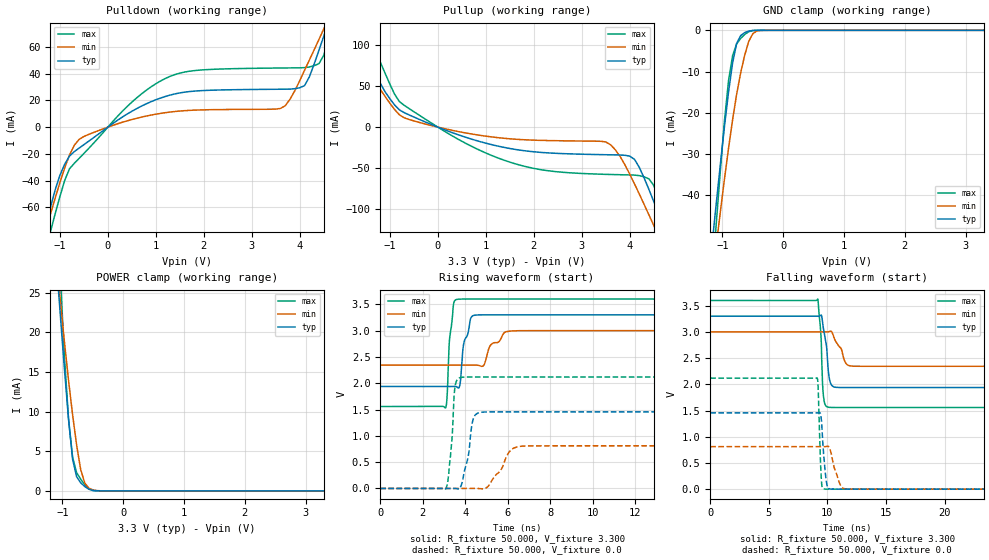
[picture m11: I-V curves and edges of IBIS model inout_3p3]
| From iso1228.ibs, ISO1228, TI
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|   Model inout_3p3
[Model] inout_3p3
Model_type I/O
Vinl =  0.990V
Vinh =  2.310V
Polarity   Non-Inverting
Enable   Active-High
Vmeas = 1.65
Vref = 0
Cref = 15pF
Rref = 1000
C_comp   0.978pF   1.050pF   0.889pF
[Model Spec]
Vinh   2.310V   2.100V   2.520V
Vinl   0.990V   0.900V   1.080V
[Temperature Range]   27.000   0.150k   -40.000
[Voltage Range]   3.300V   3.000V   3.600V
[Pullup Reference]   3.300V   3.000V   3.600V
[Pulldown Reference]   0.0V   0.0V   0.0V
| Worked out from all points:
|   slope of the pulldown table from 0 to 0.495 V, typ, clamps not added: 42.2 ohm
|   slope of the pullup table from 0 to 0.495 V, typ, clamps not added: 46.1 ohm
|   GND clamp passes 1 mA (typ) near -0.68 V on its own axis
|   POWER clamp passes 1 mA (typ) near -0.70 V on its own axis
|   rising waveform, R_fixture 50.000, V_fixture 3.300: 20-80 % time 356ps typ, 720ps min, 207ps max; typ from 1.94 V to 3.3 V
|   rising waveform, R_fixture 50.000, V_fixture 0.0: 20-80 % time 354ps typ, 726ps min, 215ps max; typ from 0 V to 1.46 V
|   falling waveform, R_fixture 50.000, V_fixture 3.300: 20-80 % time 412ps typ, 821ps min, 243ps max; typ from 3.3 V to 1.94 V
|   falling waveform, R_fixture 50.000, V_fixture 0.0: 20-80 % time 293ps typ, 603ps min, 185ps max; typ from 1.46 V to 0 V
[Pulldown]
|Voltage   I(typ)   I(min)   I(max)
-3.3V     -447.8mA   -372.8mA   -654.4mA
-1.3V     -74.39mA   -77.85mA   -94.82mA
-1.2V     -60.33mA   -65.41mA   -78.6mA
-900mV    -27.72mA   -30.46mA   -39.85mA
-600mV    -15.68mA   -9.201mA   -23.38mA
500mV     11.84mA    5.676mA    18.66mA
1.3V      23.95mA    11.27mA    37.96mA
3.6V      28.3mA     13.97mA    44.16mA
4.1V      31.01mA    42.51mA    44.42mA
4.5V      67.87mA    73.32mA    53.59mA
4.7V      89mA       89.09mA    81.73mA
6.6V      358.2mA    289.3mA    493.9mA
[Pullup]
|Voltage   I(typ)   I(min)   I(max)
-3.3V     356.7mA    258.7mA    567mA
-2.1V     161.1mA    122.4mA    246.9mA
-1.8V     121.5mA    96.5mA     180.5mA
-1.5V     87.45mA    71.23mA    126mA
-700mV    17.66mA    11.4mA     26.61mA
1.4V      -24.96mA   -13.72mA   -40.75mA
3.5V      -33.67mA   -18.07mA   -57.65mA
4.1V      -39.42mA   -69.47mA   -58.55mA
4.4V      -76.17mA   -107.2mA   -63.21mA
4.6V      -105.6mA   -132.9mA   -86.69mA
4.8V      -135.9mA   -159mA     -125.7mA
6.6V      -482.2mA   -443.3mA   -617.5mA
[GND_clamp]
|Voltage   I(typ)   I(min)   I(max)
-3.3V     -446.5mA   -372.3mA   -652.2mA
-1.167V   -51.36mA   -60.11mA   -59.79mA
-1.1V     -41.74mA   -51.92mA   -46.53mA
-1.033V   -32.37mA   -43.89mA   -33.74mA
-967mV    -23.36mA   -36.1mA    -21.98mA
-900mV    -15.01mA   -28.65mA   -12.25mA
-833mV    -7.919mA   -21.71mA   -6.137mA
-767mV    -3.23mA    -15.56mA   -3.327mA
-633mV    -537.4uA   -5.994mA   -992.5uA
-500mV    -36.13uA   -809.1uA   -56.28uA
-367mV    -1.312uA   -33.13uA   -1.236uA
3.3V      0A         0A         0A
[POWER_clamp]
|Voltage   I(typ)   I(min)   I(max)
-3.3V     327.5mA    237.7mA    524.4mA
-1.1V     28.87mA    29.08mA    37.17mA
-1.033V   22.02mA    23.87mA    26.91mA
-967mV    15.37mA    18.79mA    16.96mA
-900mV    9.079mA    13.99mA    9.126mA
-833mV    4.017mA    9.616mA    4.268mA
-767mV    1.792mA    5.817mA    2.311mA
-700mV    1.03mA     2.71mA     1.49mA
-633mV    556.9uA    1.007mA    803.4uA
-567mV    225.9uA    363.5uA    292.8uA
-300mV    7.304uA    7.368uA    10.1uA
3.3V      0A         0A         775.8nA
[Ramp]
| variable   typ   min   max
dV/dt_r   0.873/0.354n   0.487/0.726n   1.271/0.213n
dV/dt_f   0.817/0.414n   0.394/0.818n   1.225/0.244n
R_load = 50.000
[Rising Waveform]
R_fixture= 50.000
V_fixture= 3.300
V_fixture_min= 3.000
V_fixture_max= 3.600
|time   V(typ)   V(min)   V(max)
0s        1.938V     2.344V     1.558V
3.08ns    1.938V     2.344V     1.536V
3.15ns    1.938V     2.344V     1.809V
3.25ns    1.938V     2.344V     2.804V
3.43ns    1.939V     2.344V     3.455V
3.7ns     1.913V     2.344V     3.598V
3.94ns    2.78V      2.344V     3.6V
4.6ns     3.298V     2.342V     3.6V
6.49ns    3.3V       2.998V     3.6V
100ns     3.3V       3V         3.6V
[Rising Waveform]
R_fixture= 50.000
V_fixture= 0.0
V_fixture_min= 0.0
V_fixture_max= 0.0
|time   V(typ)   V(min)   V(max)
0s        258.3nV    99.06nV    1.22nV
3.08ns    1.462uV    99.06nV    -5.843mV
3.3ns     -36.21uV   95.06nV    611.5mV
3.53ns    798uV      169nV      1.972V
3.9ns     207.8mV    -2.457uV   2.116V
4.37ns    1.322V     198uV      2.118V
4.94ns    1.453V     187.2uV    2.118V
6.15ns    1.455V     733.5mV    2.118V
7.03ns    1.455V     809.6mV    2.118V
100ns     1.455V     810.9mV    2.118V
[Falling Waveform]
R_fixture= 50.000
V_fixture= 3.300
V_fixture_min= 3.000
V_fixture_max= 3.600
|time   V(typ)   V(min)   V(max)
0s        3.3V       3V         3.6V
9.17ns    3.3V       3V         3.626V
9.44ns    3.319V     3V         2.956V
9.57ns    3.208V     3V         2.064V
9.65ns    3.074V     3V         1.79V
9.92ns    2.727V     2.999V     1.577V
10.18ns   2.089V     3.009V     1.561V
11.59ns   1.938V     2.396V     1.558V
12.24ns   1.938V     2.345V     1.558V
100ns     1.938V     2.344V     1.558V
[Falling Waveform]
R_fixture= 50.000
V_fixture= 0.0
V_fixture_min= 0.0
V_fixture_max= 0.0
|time   V(typ)   V(min)   V(max)
0s        1.455V     810.9mV    2.118V
9.12ns    1.455V     810.9mV    2.12V
9.2ns     1.455V     810.9mV    1.974V
9.39ns    1.445V     810.9mV    610.3mV
9.49ns    1.3V       810.7mV    148.6mV
9.78ns    402.3mV    810.8mV    1.903mV
10.08ns   17.47mV    814.8mV    339uV
11.07ns   102.2uV    95.09mV    28.8uV
11.8ns    32.17uV    1.27mV     6.031uV
100ns     27.81nV    117.9nV    35.37nV
